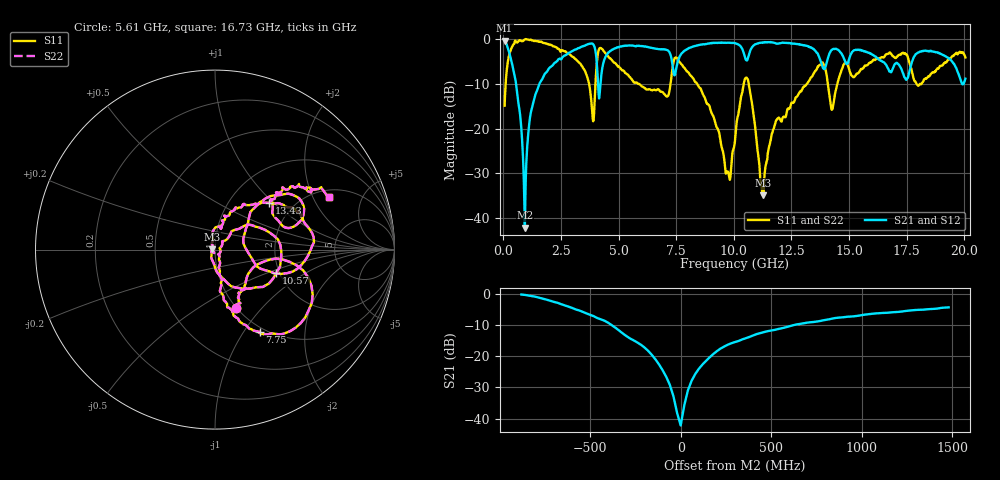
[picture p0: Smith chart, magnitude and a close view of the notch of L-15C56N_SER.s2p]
#	mhz	s	ma	r	50
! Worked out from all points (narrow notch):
!   1001 points, 50 MHz to 20.05 GHz, reference 50 ohm
!   highest |S21| = -0.26 dB at 50 MHz (marker M1); lowest = -42.2 dB at 930 MHz (marker M2)
!   notch at M2: 39.6 dB deep, 248 MHz wide at half that depth
!   lowest |S11| = -34.9 dB at 11.25 GHz (marker M3), VSWR 1.04, Z = 48.3 + j0.182 ohm
!   |S11| at or under -10 dB: 5.9 GHz to 7.252 GHz (1.352 GHz wide, 20.6 % of centre); 8.415 GHz to 10.43 GHz (2.011 GHz wide, 21.4 % of centre); 10.65 GHz to 13.16 GHz (2.518 GHz wide, 21.1 % of centre)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
!   |S22| runs from -34.9 to 0.1 dB; largest |S21 - S12| = 0
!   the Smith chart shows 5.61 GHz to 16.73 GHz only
!   S11 on the Smith chart (normalised r, x): 5.61 GHz: 1.00, -0.74; 7.75 GHz: 0.94, -1.18; 10.57 GHz: 1.92, -0.58; 13.43 GHz: 1.51, +0.94; 16.73 GHz: 2.34, +2.67
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50  0.1808 76.7  0.9707 -9.7  0.9707 -9.7  0.1808 76.7
550  0.9361 17.6  0.3125 -69.2  0.3125 -69.2  0.9361 17.6
930  0.9998 -6.7  0.00777 5.0  0.00777 5.0  0.9998 -6.7
1550  0.9522 -23.7  0.3126 66.3  0.3126 66.3  0.9522 -23.7
3390  0.5093 -62.5  0.8254 23.6  0.8254 23.6  0.5093 -62.5
3870  0.135 -49.1  0.8948 -2.9  0.8948 -2.9  0.135 -49.1
4190  0.8026 -19.9  0.2716 27.9  0.2716 27.9  0.8026 -19.9
5610  0.3465 -70.0  0.8555 6.5  0.8555 6.5  0.3465 -70.0
6730  0.2763 -52.8  0.7801 -5.3  0.7801 -5.3  0.2763 -52.8
7750  0.5208 -61.6  0.7044 12.4  0.7044 12.4  0.5208 -61.6
9750  0.03286 -19.8  0.9206 -15.1  0.9206 -15.1  0.03286 -19.8
10050  0.07354 42.2  0.9099 -20.5  0.9099 -20.5  0.07354 42.2
10570  0.3653 -20.8  0.5814 -14.2  0.5814 -14.2  0.3653 -20.8
11250  0.01789 174.0  0.9166 -16.9  0.9166 -16.9  0.01789 174.0
11830  0.1231 88.9  0.9012 -25.4  0.9012 -25.4  0.1231 88.9
13390  0.3837 42.8  0.8023 -47.3  0.8023 -47.3  0.3837 42.8
13430  0.3988 40.8  0.7881 -48.0  0.7881 -48.0  0.3988 40.8
14270  0.1641 16.8  0.7696 -29.8  0.7696 -29.8  0.1641 16.8
14810  0.5423 32.9  0.5831 -46.7  0.5831 -46.7  0.5423 32.9
16730  0.6986 24.7  0.4513 -51.3  0.4513 -51.3  0.6986 24.7
17990  0.3046 5.9  0.712 -25.7  0.712 -25.7  0.3046 5.9
20050  0.6296 -25.3  0.3634 -36.3  0.3634 -36.3  0.6296 -25.3
